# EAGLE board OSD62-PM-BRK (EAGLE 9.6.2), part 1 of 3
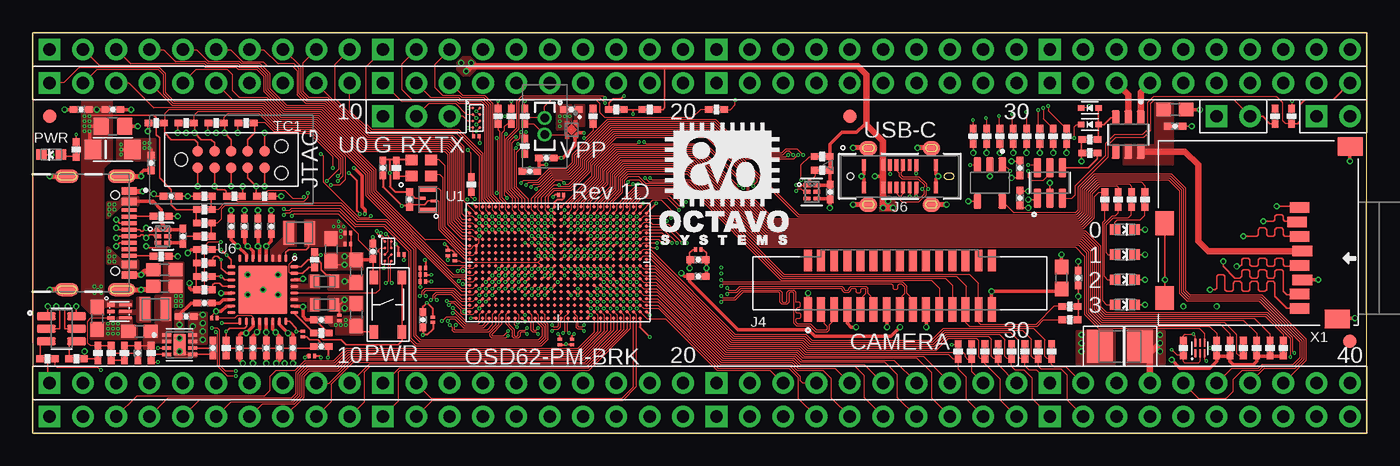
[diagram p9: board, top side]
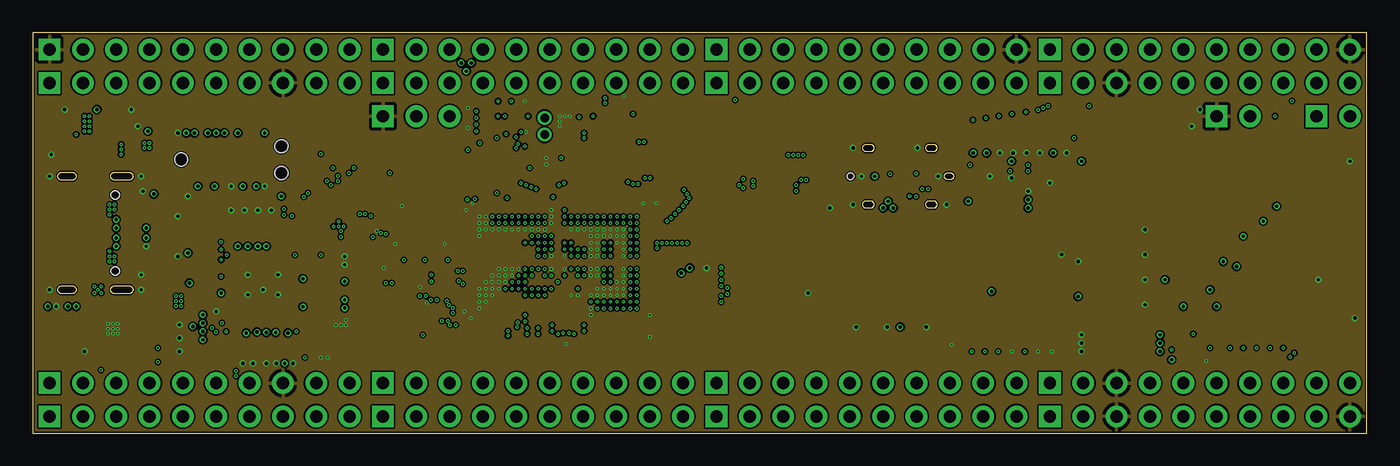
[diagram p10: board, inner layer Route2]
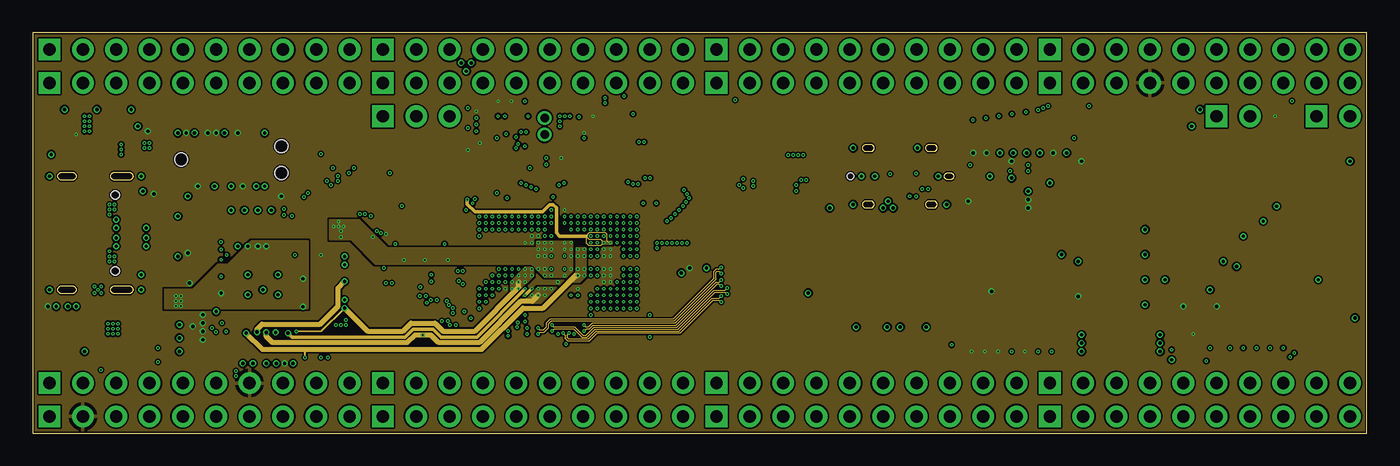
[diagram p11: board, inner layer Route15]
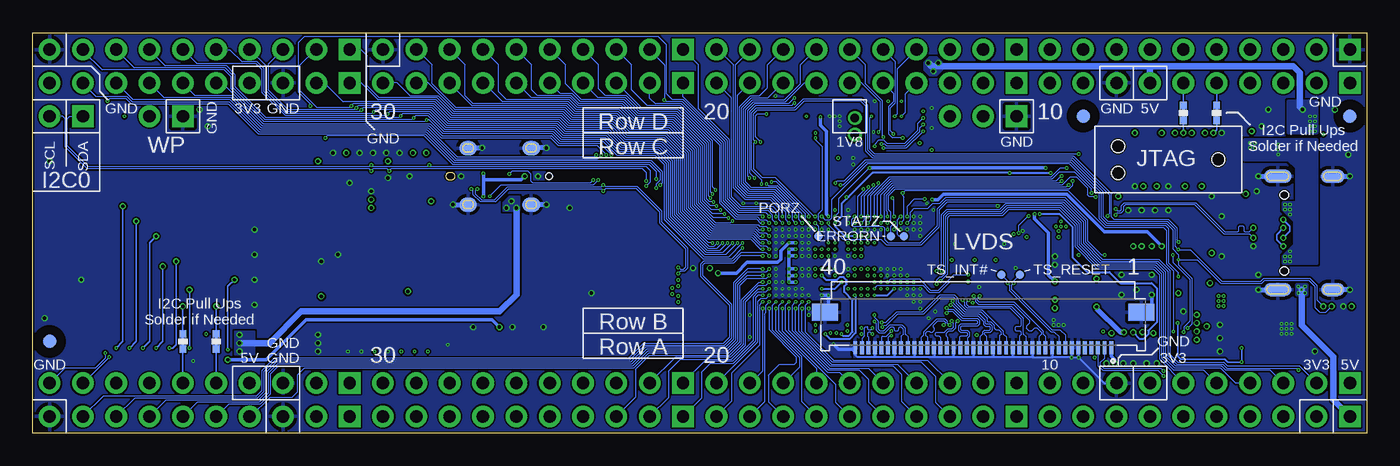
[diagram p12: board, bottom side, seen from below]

Size 101.6 x 30.48 mm. Coordinates in mm from the lower left corner, seen from the top.
Outline: 0,0 101.6,0 101.6,30.48 0,30.48 0,0
Copper layers (1+2*15+16): Top 0.035mm / dielectric 0.23mm / Route2 0.035mm / dielectric 0.93mm / Route15 0.035mm / dielectric 0.23mm / Bottom 0.035mm
Design rules "OSD32MP15x-BRK_Board_4lyr *": minimum track width 3mil, minimum drill 4mil, track to track 3mil, track to pad 3mil, pad to pad 3mil, via to via 3mil, smd to smd 3mil, copper to edge 5mil, drill to drill 4mil, minimum pad ring 3mil, minimum via ring 3mil, stop-mask expansion 3mil, vias tented up to drill 25mil, thermal gap 10mil

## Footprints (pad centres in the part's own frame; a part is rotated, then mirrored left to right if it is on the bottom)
C0201 = smd 0.23 x 0.34: 1 -0.205,0; 2 0.205,0
C0402 = smd 0.61 x 0.508: 1 -0.559,0; 2 0.559,0
B/3528-21R = smd 1.95 x 2.5: + 1.525,0; - -1.525,0
C0603 = smd 1.1 x 1: 1 -0.85,0; 2 0.85,0
C0805 = smd 1.143 x 1.27: 1 -0.889,0; 2 0.889,0
EIA-STD = smd 0.787 x 0.787: 1 -0.749,0; 2 0.749,0
RB520S30T1G = smd 0.48 x 0.4: ANODE 0.66,0; CATHODE -0.66,0
SOD-123FL = smd 1.25 x 1.5: A 1.5,0; C -1.5,0
FIDUCIAL_40MIL = smd 1.016 x 1.016: P$1 0,0
H1X2-1.27 = drill 0.65 pad 1.05: 1 -0.635,0; 2 0.635,0
H1X2-2.54 = drill 0.94 pad 1.651 square: 1 0,1.27 | drill 0.94 pad 1.651: 2 0,-1.27
TE_1-1734248-5 = smd 0.6 x 1.85: 1 -7,-2.025; 2 -6,-2.025; 3 -5,-2.025; 4 -4,-2.025; 5 -3,-2.025; 6 -2,-2.025; 7 -1,-2.025; 8 0,-2.025; 9 1,-2.025; 10 2,-2.025; 11 3,-2.025; 12 4,-2.025; 13 5,-2.025; 14 6,-2.025; 15 7,-2.025 | smd 0.6 x 1.65: 1_1 -7,1.725; 2_1 -6,1.725; 3_1 -5,1.725; 4_1 -4,1.725; 5_1 -3,1.725; 6_1 -2,1.725; 7_1 -1,1.725; 8_1 0,1.725; 9_1 1,1.725; 10_1 2,1.725; 11_1 3,1.725; 12_1 4,1.725; 13_1 5,1.725; 14_1 6,1.725; 15_1 7,1.725
GCT_USB4105-GF-A = smd 0.6 x 1.15: A1_B12 -3.2,4.755; A4_B9 -2.4,4.755; B1_A12 3.2,4.755; B4_A9 2.4,4.755 | smd 0.3 x 1.15: A5 -1.25,4.755; A6 -0.25,4.755; A7 0.25,4.755; A8 1.25,4.755; B5 1.75,4.755; B6 0.75,4.755; B7 -0.75,4.755; B8 -1.75,4.755 | smd 1 x 2.1 bottom: SH1_B -4.32,4.18; SH2_B 4.32,4.18 | smd 1 x 2.1: SH1_T -4.32,4.18; SH2_T 4.32,4.18 | smd 1 x 1.8 bottom: SH3_B 4.32,0; SH4_B -4.32,0 | smd 1 x 1.8: SH3_T 4.32,0; SH4_T -4.32,0 | hole 0.65: 2.89,3.68; -2.89,3.68
MOLEX_2171820001 = smd 0.3 x 0.87: A1 -2.75,0.865; A4 -1.25,0.865; A5 -0.75,0.865; A6 -0.25,0.865; A7 0.25,0.865; A8 0.75,0.865; A9 1.25,0.865; A12 2.75,0.865; B1 2.75,-0.865; B4 1.25,-0.865; B5 0.75,-0.865; B6 0.25,-0.865; B7 -0.25,-0.865; B8 -0.75,-0.865; B9 -1.25,-0.865; B12 -2.75,-0.865 | smd 1.35 x 1.1 bottom: SH_B_1 -2.4,2.15; SH_B_2 2.4,2.15; SH_B_3 2.4,-2.15; SH_B_4 -2.4,-2.15 | smd 1.35 x 1.1: SH_T_1 -2.4,2.15; SH_T_2 2.4,2.15; SH_T_3 2.4,-2.15; SH_T_4 -2.4,-2.15 | hole 0.52: -3.75,0
MOLEX_505110-4091 = smd 0.3 x 1: 1 -9.75,2.425; 2 -9.25,2.425; 3 -8.75,2.425; 4 -8.25,2.425; 5 -7.75,2.425; 6 -7.25,2.425; 7 -6.75,2.425; 8 -6.25,2.425; 9 -5.75,2.425; 10 -5.25,2.425; 11 -4.75,2.425; 12 -4.25,2.425; 13 -3.75,2.425; 14 -3.25,2.425; 15 -2.75,2.425; 16 -2.25,2.425; 17 -1.75,2.425; 18 -1.25,2.425; 19 -0.75,2.425; 20 -0.25,2.425; 21 0.25,2.425; 22 0.75,2.425; 23 1.25,2.425; 24 1.75,2.425; 25 2.25,2.425; 26 2.75,2.425; 27 3.25,2.425; 28 3.75,2.425; 29 4.25,2.425; 30 4.75,2.425; 31 5.25,2.425; 32 5.75,2.425; 33 6.25,2.425; 34 6.75,2.425; 35 7.25,2.425; 36 7.75,2.425; 37 8.25,2.425; 38 8.75,2.425; 39 9.25,2.425; 40 9.75,2.425 | smd 2 x 1.3: S1 -12.05,-0.275; S2 12.05,-0.275
H1X3-2.54 = drill 0.94 pad 1.651 square: 1 0,2.54 | drill 0.94 pad 1.651: 2 0,0; 3 0,-2.54
H1X40-2.54 = drill 0.94 pad 1.651 square: 1 0,49.53; 11 0,24.13; 21 0,-1.27; 31 0,-26.67 | drill 0.94 pad 1.651: 2 0,46.99; 3 0,44.45; 4 0,41.91; 5 0,39.37; 6 0,36.83; 7 0,34.29; 8 0,31.75; 9 0,29.21; 10 0,26.67; 12 0,21.59; 13 0,19.05; 14 0,16.51; 15 0,13.97; 16 0,11.43; 17 0,8.89; 18 0,6.35; 19 0,3.81; 20 0,1.27; 22 0,-3.81; 23 0,-6.35; 24 0,-8.89; 25 0,-11.43; 26 0,-13.97; 27 0,-16.51; 28 0,-19.05; 29 0,-21.59; 30 0,-24.13; 32 0,-29.21; 33 0,-31.75; 34 0,-34.29; 35 0,-36.83; 36 0,-39.37; 37 0,-41.91; 38 0,-44.45; 39 0,-46.99; 40 0,-49.53
L0806 = smd 0.8 x 1.8: 1 -0.8,0; 2 0.8,0
L0603 = smd 0.7 x 1: 1 -0.75,0; 2 0.75,0
R0402 = smd 0.61 x 0.508: 1 -0.559,0; 2 0.559,0
TACT4.2MM = smd 1.05 x 0.65: P$1 -2.075,1.075; P$2 2.075,1.075; P$3 -2.075,-1.075; P$4 2.075,-1.075
TC2050-IDC-NL = smd 0.787 x 0.787: 1 -2.54,-0.635; 2 -1.27,-0.635; 3 0,-0.635; 4 1.27,-0.635; 5 2.54,-0.635; 6 2.54,0.635; 7 1.27,0.635; 8 0,0.635; 9 -1.27,0.635; 10 -2.54,0.635 | hole 0.991: -3.81,0; 3.81,1.016; 3.81,-1.016
TP_B0,65 = smd 0.635 x 0.635: TP 0,0
BGA-500-9X14MM = smd 0.25 x 0.25: A2 -6.25,4.25; A3 -5.75,4.25; A4 -5.25,4.25; A5 -4.75,4.25; A6 -4.25,4.25; A7 -3.75,4.25; A8 -3.25,4.25; A9 -2.75,4.25; A10 -2.25,4.25; A11 -1.75,4.25; A12 -1.25,4.25; A13 -0.75,4.25; A14 -0.25,4.25; A15 0.25,4.25; A16 0.75,4.25; A17 1.25,4.25; A18 1.75,4.25; A19 2.25,4.25; A20 2.75,4.25; A21 3.25,4.25; A22 3.75,4.25; A23 4.25,4.25; A24 4.75,4.25; A25 5.25,4.25; A26 5.75,4.25; A27 6.25,4.25; B1 -6.75,3.75; B2 -6.25,3.75; B3 -5.75,3.75; B4 -5.25,3.75; B5 -4.75,3.75; B6 -4.25,3.75; B7 -3.75,3.75; B8 -3.25,3.75; B9 -2.75,3.75; B10 -2.25,3.75; B11 -1.75,3.75; B12 -1.25,3.75; B13 -0.75,3.75; B14 -0.25,3.75; B15 0.25,3.75; B16 0.75,3.75; B17 1.25,3.75; B18 1.75,3.75; B19 2.25,3.75; B20 2.75,3.75; B21 3.25,3.75; B22 3.75,3.75; B23 4.25,3.75; B24 4.75,3.75; B25 5.25,3.75; B26 5.75,3.75; B27 6.25,3.75; B28 6.75,3.75; C1 -6.75,3.25; C2 -6.25,3.25; C3 -5.75,3.25; C4 -5.25,3.25; C5 -4.75,3.25; C6 -4.25,3.25; C7 -3.75,3.25; C8 -3.25,3.25; C9 -2.75,3.25; C10 -2.25,3.25; C11 -1.75,3.25; C12 -1.25,3.25; C13 -0.75,3.25; C14 -0.25,3.25; C15 0.25,3.25; C16 0.75,3.25; C17 1.25,3.25; C18 1.75,3.25; C19 2.25,3.25; C20 2.75,3.25; C21 3.25,3.25; C22 3.75,3.25; C23 4.25,3.25; C24 4.75,3.25; C25 5.25,3.25; C26 5.75,3.25; C27 6.25,3.25; C28 6.75,3.25; D1 -6.75,2.75; D2 -6.25,2.75; D3 -5.75,2.75; D4 -5.25,2.75; D5 -4.75,2.75; D6 -4.25,2.75; D7 -3.75,2.75; D8 -3.25,2.75; D9 -2.75,2.75; D10 -2.25,2.75; D11 -1.75,2.75; D12 -1.25,2.75; D13 -0.75,2.75; D14 -0.25,2.75; D15 0.25,2.75; D16 0.75,2.75; D17 1.25,2.75; D18 1.75,2.75; D19 2.25,2.75; D20 2.75,2.75; D21 3.25,2.75; D22 3.75,2.75; D23 4.25,2.75; D24 4.75,2.75; D25 5.25,2.75; D26 5.75,2.75; D27 6.25,2.75; D28 6.75,2.75; E1 -6.75,2.25; E2 -6.25,2.25; E3 -5.75,2.25; E4 -5.25,2.25; E5 -4.75,2.25; E6 -4.25,2.25; E7 -3.75,2.25; E8 -3.25,2.25; E9 -2.75,2.25; E10 -2.25,2.25; E11 -1.75,2.25; E12 -1.25,2.25; E13 -0.75,2.25; E14 -0.25,2.25; E15 0.25,2.25; E16 0.75,2.25; E17 1.25,2.25; E18 1.75,2.25; E19 2.25,2.25; E20 2.75,2.25; E21 3.25,2.25; E22 3.75,2.25; E23 4.25,2.25; E24 4.75,2.25; E25 5.25,2.25; E26 5.75,2.25; E27 6.25,2.25; E28 6.75,2.25; F1 -6.75,1.75; F2 -6.25,1.75; F3 -5.75,1.75; F4 -5.25,1.75; F5 -4.75,1.75; F6 -4.25,1.75; F7 -3.75,1.75; F8 -3.25,1.75; F9 -2.75,1.75; F10 -2.25,1.75; F11 -1.75,1.75; F12 -1.25,1.75; F13 -0.75,1.75; F14 -0.25,1.75; F15 0.25,1.75; F16 0.75,1.75; F17 1.25,1.75; F18 1.75,1.75; F19 2.25,1.75; F20 2.75,1.75; F21 3.25,1.75; F22 3.75,1.75; F23 4.25,1.75; F24 4.75,1.75; F25 5.25,1.75; F26 5.75,1.75; F27 6.25,1.75; F28 6.75,1.75; G1 -6.75,1.25; G2 -6.25,1.25; G3 -5.75,1.25; G4 -5.25,1.25; G5 -4.75,1.25; G6 -4.25,1.25; G7 -3.75,1.25; G8 -3.25,1.25; G9 -2.75,1.25; G10 -2.25,1.25; G11 -1.75,1.25; G12 -1.25,1.25; G13 -0.75,1.25; G14 -0.25,1.25; G15 0.25,1.25; G16 0.75,1.25; G17 1.25,1.25; G18 1.75,1.25; G19 2.25,1.25; G20 2.75,1.25; G21 3.25,1.25; G22 3.75,1.25; G23 4.25,1.25; G24 4.75,1.25; G25 5.25,1.25; G26 5.75,1.25; G27 6.25,1.25; G28 6.75,1.25; H1 -6.75,0.75; H2 -6.25,0.75; H3 -5.75,0.75; H4 -5.25,0.75; H5 -4.75,0.75; H6 -4.25,0.75; H7 -3.75,0.75; H8 -3.25,0.75; H9 -2.75,0.75; H10 -2.25,0.75; H11 -1.75,0.75; H12 -1.25,0.75; H13 -0.75,0.75; H14 -0.25,0.75; H15 0.25,0.75; H16 0.75,0.75; H17 1.25,0.75; H18 1.75,0.75; H19 2.25,0.75; H20 2.75,0.75; H21 3.25,0.75; H22 3.75,0.75; H23 4.25,0.75; H24 4.75,0.75; H25 5.25,0.75; H26 5.75,0.75; H27 6.25,0.75; H28 6.75,0.75; J1 -6.75,0.25; J2 -6.25,0.25; J3 -5.75,0.25; J4 -5.25,0.25; J5 -4.75,0.25; J6 -4.25,0.25; J7 -3.75,0.25; J8 -3.25,0.25; J9 -2.75,0.25; J10 -2.25,0.25; J11 -1.75,0.25; J12 -1.25,0.25; J13 -0.75,0.25; J14 -0.25,0.25; J15 0.25,0.25; J16 0.75,0.25; J17 1.25,0.25; J18 1.75,0.25; J19 2.25,0.25; J20 2.75,0.25; J21 3.25,0.25; J22 3.75,0.25; J23 4.25,0.25; J24 4.75,0.25; J25 5.25,0.25; J26 5.75,0.25; J27 6.25,0.25; J28 6.75,0.25; K1 -6.75,-0.25; K2 -6.25,-0.25; K3 -5.75,-0.25; K4 -5.25,-0.25; K5 -4.75,-0.25; K6 -4.25,-0.25; K7 -3.75,-0.25; K8 -3.25,-0.25; K9 -2.75,-0.25; K10 -2.25,-0.25; K11 -1.75,-0.25; K12 -1.25,-0.25; K13 -0.75,-0.25; K14 -0.25,-0.25; K15 0.25,-0.25; K16 0.75,-0.25; K17 1.25,-0.25; K18 1.75,-0.25; K19 2.25,-0.25; K20 2.75,-0.25; K21 3.25,-0.25; K22 3.75,-0.25; K23 4.25,-0.25; K24 4.75,-0.25; K25 5.25,-0.25; K26 5.75,-0.25; K27 6.25,-0.25; K28 6.75,-0.25; L1 -6.75,-0.75; L2 -6.25,-0.75; L3 -5.75,-0.75; L4 -5.25,-0.75; L5 -4.75,-0.75; L6 -4.25,-0.75; L7 -3.75,-0.75; L8 -3.25,-0.75; L9 -2.75,-0.75; L10 -2.25,-0.75; L11 -1.75,-0.75; L12 -1.25,-0.75; L13 -0.75,-0.75; L14 -0.25,-0.75; L15 0.25,-0.75; L16 0.75,-0.75; L17 1.25,-0.75; L18 1.75,-0.75; L19 2.25,-0.75; L20 2.75,-0.75; L21 3.25,-0.75; L22 3.75,-0.75; L23 4.25,-0.75; L24 4.75,-0.75; L25 5.25,-0.75; L26 5.75,-0.75; L27 6.25,-0.75; L28 6.75,-0.75; M1 -6.75,-1.25; M2 -6.25,-1.25; M3 -5.75,-1.25; M4 -5.25,-1.25; M5 -4.75,-1.25; M6 -4.25,-1.25; M7 -3.75,-1.25; M8 -3.25,-1.25; M9 -2.75,-1.25; M10 -2.25,-1.25; M11 -1.75,-1.25; M12 -1.25,-1.25; M13 -0.75,-1.25; M14 -0.25,-1.25; M15 0.25,-1.25; M16 0.75,-1.25; M17 1.25,-1.25; M18 1.75,-1.25; M19 2.25,-1.25; M20 2.75,-1.25; M21 3.25,-1.25; M22 3.75,-1.25; M23 4.25,-1.25; M24 4.75,-1.25; M25 5.25,-1.25; M26 5.75,-1.25; M27 6.25,-1.25; M28 6.75,-1.25; N1 -6.75,-1.75; N2 -6.25,-1.75; N3 -5.75,-1.75; N4 -5.25,-1.75; N5 -4.75,-1.75; N6 -4.25,-1.75; N7 -3.75,-1.75; N8 -3.25,-1.75; N9 -2.75,-1.75; N10 -2.25,-1.75; N11 -1.75,-1.75; N12 -1.25,-1.75; N13 -0.75,-1.75; N14 -0.25,-1.75; N15 0.25,-1.75; N16 0.75,-1.75; N17 1.25,-1.75; N18 1.75,-1.75; N19 2.25,-1.75; N20 2.75,-1.75; N21 3.25,-1.75; N22 3.75,-1.75; N23 4.25,-1.75; N24 4.75,-1.75; N25 5.25,-1.75; N26 5.75,-1.75; N27 6.25,-1.75; N28 6.75,-1.75; P1 -6.75,-2.25; P2 -6.25,-2.25; P3 -5.75,-2.25; P4 -5.25,-2.25; P5 -4.75,-2.25; P6 -4.25,-2.25; P7 -3.75,-2.25; P8 -3.25,-2.25; P9 -2.75,-2.25; P10 -2.25,-2.25; P11 -1.75,-2.25; P12 -1.25,-2.25; P13 -0.75,-2.25; P14 -0.25,-2.25; P15 0.25,-2.25; P16 0.75,-2.25; P17 1.25,-2.25; P18 1.75,-2.25; P19 2.25,-2.25; P20 2.75,-2.25; P21 3.25,-2.25; P22 3.75,-2.25; P23 4.25,-2.25; P24 4.75,-2.25; P25 5.25,-2.25; P26 5.75,-2.25; P27 6.25,-2.25; P28 6.75,-2.25; R1 -6.75,-2.75; R2 -6.25,-2.75; R3 -5.75,-2.75; R4 -5.25,-2.75; R5 -4.75,-2.75; R6 -4.25,-2.75; R7 -3.75,-2.75; R8 -3.25,-2.75; R9 -2.75,-2.75; R10 -2.25,-2.75; R11 -1.75,-2.75; R12 -1.25,-2.75; R13 -0.75,-2.75; R14 -0.25,-2.75; R15 0.25,-2.75; R16 0.75,-2.75; R17 1.25,-2.75; R18 1.75,-2.75; R19 2.25,-2.75; R20 2.75,-2.75; R21 3.25,-2.75; R22 3.75,-2.75; R23 4.25,-2.75; R24 4.75,-2.75; R25 5.25,-2.75; R26 5.75,-2.75; R27 6.25,-2.75; R28 6.75,-2.75; T1 -6.75,-3.25; T2 -6.25,-3.25; T3 -5.75,-3.25; T4 -5.25,-3.25; T5 -4.75,-3.25; T6 -4.25,-3.25; T7 -3.75,-3.25; T8 -3.25,-3.25; T9 -2.75,-3.25; T10 -2.25,-3.25; T11 -1.75,-3.25; T12 -1.25,-3.25; T13 -0.75,-3.25; T14 -0.25,-3.25; T15 0.25,-3.25; T16 0.75,-3.25; T17 1.25,-3.25; T18 1.75,-3.25; T19 2.25,-3.25; T20 2.75,-3.25; T21 3.25,-3.25; T22 3.75,-3.25; T23 4.25,-3.25; T24 4.75,-3.25; T25 5.25,-3.25; T26 5.75,-3.25; T27 6.25,-3.25; T28 6.75,-3.25; U1 -6.75,-3.75; U2 -6.25,-3.75; U3 -5.75,-3.75; U4 -5.25,-3.75; U5 -4.75,-3.75; U6 -4.25,-3.75; U7 -3.75,-3.75; U8 -3.25,-3.75; U9 -2.75,-3.75; U10 -2.25,-3.75; U11 -1.75,-3.75; U12 -1.25,-3.75; U13 -0.75,-3.75; U14 -0.25,-3.75; U15 0.25,-3.75; U16 0.75,-3.75; U17 1.25,-3.75; U18 1.75,-3.75; U19 2.25,-3.75; U20 2.75,-3.75; U21 3.25,-3.75; U22 3.75,-3.75; U23 4.25,-3.75; U24 4.75,-3.75; U25 5.25,-3.75; U26 5.75,-3.75; U27 6.25,-3.75; U28 6.75,-3.75; V2 -6.25,-4.25; V3 -5.75,-4.25; V4 -5.25,-4.25; V5 -4.75,-4.25; V6 -4.25,-4.25; V7 -3.75,-4.25; V8 -3.25,-4.25; V9 -2.75,-4.25; V10 -2.25,-4.25; V11 -1.75,-4.25; V12 -1.25,-4.25; V13 -0.75,-4.25; V14 -0.25,-4.25; V15 0.25,-4.25; V16 0.75,-4.25; V17 1.25,-4.25; V18 1.75,-4.25; V19 2.25,-4.25; V20 2.75,-4.25; V21 3.25,-4.25; V22 3.75,-4.25; V23 4.25,-4.25; V24 4.75,-4.25; V25 5.25,-4.25; V26 5.75,-4.25; V27 6.25,-4.25
DRY6 = smd 0.55 x 0.3: 1 -0.355,0.5 | smd 0.52 x 0.3: 2 -0.37,0; 3 -0.37,-0.5; 4 0.37,-0.5; 5 0.37,0; 6 0.37,0.5
DMQ0006A = smd 0.6 x 0.25: 1 -0.65,0.5; 2 -0.65,0; 3 -0.65,-0.5 | smd 1 x 0.2: 4 0.45,-0.5; 5 0.45,0; 6 0.45,0.5
SOT95P280X145-5N = smd 1.1 x 0.6: 1 -1.4,0.95; 2 -1.4,0; 3 -1.4,-0.95; 4 1.4,-0.95; 5 1.4,0.95
SON50P200X200X80-9N = smd 0.76 x 0.28: 1 -0.985,0.75; 2 -0.985,0.25; 3 -0.985,-0.25; 4 -0.985,-0.75; 5 0.985,-0.75; 6 0.985,-0.25; 7 0.985,0.25; 8 0.985,0.75 | smd 0.9 x 1.6: 9 0,0
RHB0032W = smd 0.6 x 0.25: 1 -2.4,1.75; 2 -2.4,1.25; 3 -2.4,0.75; 4 -2.4,0.25; 5 -2.4,-0.25; 6 -2.4,-0.75; 7 -2.4,-1.25; 8 -2.4,-1.75; 17 2.4,-1.75; 18 2.4,-1.25; 19 2.4,-0.75; 20 2.4,-0.25; 21 2.4,0.25; 22 2.4,0.75; 23 2.4,1.25; 24 2.4,1.75 | smd 0.25 x 0.6: 9 -1.75,-2.4; 10 -1.25,-2.4; 11 -0.75,-2.4; 12 -0.25,-2.4; 13 0.25,-2.4; 14 0.75,-2.4; 15 1.25,-2.4; 16 1.75,-2.4; 25 1.75,2.4; 26 1.25,2.4; 27 0.75,2.4; 28 0.25,2.4; 29 -0.25,2.4; 30 -0.75,2.4; 31 -1.25,2.4; 32 -1.75,2.4 | smd 3.7 x 3.7: PAD 0,0
SOT95P280X110-6N = smd 1.45 x 0.59: 1 -1.155,0.95; 2 -1.155,0; 3 -1.155,-0.95; 4 1.155,-0.95; 5 1.155,0; 6 1.155,0.95
SOT95P280X145-6N = smd 1.1 x 0.6: 1 -1.3,0.95; 2 -1.3,0; 3 -1.3,-0.95; 4 1.3,-0.95; 5 1.3,0; 6 1.3,0.95
SON35P100X100X40-6N = smd 0.6 x 0.17: 1 -0.4,0.35; 2 -0.4,0; 3 -0.4,-0.35; 4 0.4,-0.35; 5 0.4,0; 6 0.4,0.35
YZP0008 = smd 0.23 x 0.23: A1 -0.25,0.75; A2 0.25,0.75; B1 -0.25,0.25; B2 0.25,0.25; C1 -0.25,-0.25; C2 0.25,-0.25; D1 -0.25,-0.75; D2 0.25,-0.75
DQN0004A = smd 0.05 x 0.05: 1 -0.43,0.325; 2 -0.43,-0.325; 3 0.43,-0.325; 4 0.43,0.325; 5 0,0
MF-MICROSD = smd 1.4 x 1.9: G0 -6.589,7.001; G1 6.561,6.001 | smd 0.8 x 1.5: PIN1 -1.939,3.151; PIN2 -0.839,2.951; PIN3 0.261,3.151; PIN4 1.361,3.351; PIN5 2.461,3.151; PIN6 3.561,3.351; PIN7 4.661,3.151; PIN8 5.761,3.151 | smd 1.8 x 1.4: PIN9 4.961,-7.149; PIN10 -0.739,-7.149
SIT1533AI_2X1.2MM = smd 0.4 x 1.4: 1 -0.8,0; 3 0.8,0 | smd 0.2 x 0.5: 2 -0.1,-0.45; 4 0.1,0.45
QFN-4-2X1.6MM = smd 0.9 x 0.8: 1 -0.75,-0.6; 2 0.75,-0.6; 3 0.75,0.6; 4 -0.75,0.6

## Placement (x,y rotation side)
C1  0.1uF  [C0201]  30.48,8.64 90 top
C2  0.1uF  [C0201]  41.07,6.93 270 top
C3  0.1uF  [C0201]  40.23,18.14 0 top
C4  1uF  [C0402]  29.72,8.64 90 top
C5  4.7uF  [C0402]  21.97,6.6 0 top
C6  0.1uF  [C0201]  50.67,13.97 0 top
C7  0.1uF  [C0201]  23.37,8.76 270 top
C8  0.1uF  [C0201]  29.72,12.06 180 top
C9  0.1uF  [C0201]  20.57,7.54 270 top
C10  0.1uF  [C0201]  31.62,13.72 90 top
C11  0.1uF  [C0201]  24,15.24 0 top
C12  0.1uF  [C0201]  28.07,13.59 180 top
C13  0.1uF  [C0201]  32.13,13.34 90 top
C14  0.1uF  [C0201]  24,14.4 0 top
C15  0.1uF  [C0201]  29.72,12.57 180 top
C16  10uF  [C0402]  25.91,13.84 270 top
C17  0.1uF  [C0201]  21.26,5.87 0 top
C18  0.1uF  [C0201]  13.84,8.76 180 top
C19  0.1uF  [C0201]  40.16,6.93 270 top
C20  0.1uF  [C0201]  29.72,11.56 180 top
C21  2.2uF  [C0402]  37.85,19.94 0 top
C22  2.2uF  [C0402]  50.67,13.21 0 top
C23  2.2uF  [C0402]  50.67,11.94 0 top
C24  0.1uF  [C0402]  60.73,18.36 270 top
C25  220uF  [B/3528-21R]  82.8,6.6 0 top
C26  0.1uF  [C0402]  75.18,17.91 90 top
C27  10uF  [C0603]  4.9,8.74 270 top
C28  DNP  [C0402]  13.72,6.48 270 top
C29  0.1uF  [C0402]  11.68,8.89 180 top
C30  120pF  [C0402]  8,6.1 90 top
C31  10uF  [C0603]  10.03,11.18 180 top
C32  10uF  [C0603]  10.03,12.45 180 top
C33  10uF  [C0603]  8.13,7.75 180 top
C34  0.1uF  [C0402]  10.54,18.03 0 top
C35  0.1uF  [C0402]  75.18,20.19 270 top
C36  0.1uF  [C0402]  79.63,11.81 90 top
C37  10uF  [C0603]  78.36,11.81 90 top
C38  10uF  [C0402]  16.76,6.48 270 top
C39  10uF  [C0402]  18.8,6.48 270 top
C40  10uF  [C0402]  16.13,15.75 90 top
C41  2.2uF  [C0402]  13.08,9.91 180 top
C42  10uF  [C0402]  15.11,15.75 90 top
C43  10uF  [C0402]  15.75,6.48 270 top
C44  10uF  [C0402]  17.78,6.48 270 top
C45  10uF  [C0402]  19.81,6.48 270 top
C46  0.1uF  [C0402]  28.7,17.78 270 top
C47  47uF  [C0603]  24.64,9.02 270 top
C48  22uF  [C0402]  21.97,8.64 0 top
C49  47uF  [C0603]  24.64,12.32 90 top
C50  0.1uF  [C0402]  11.43,14.99 270 top
C51  10uF  [C0402]  17.14,15.75 90 top
C52  22uF  [C0402]  18.16,15.75 90 top
C53  47uF  [C0603]  22.73,13.97 270 top
C54  0.1uF  [C0402]  26.67,20.19 270 top
C55  0.1uF  [C0402]  6.1,24.64 0 top
C56  47uF  [C0805]  6.1,23.37 0 top
C57  10uF  [C0603]  87,24.64 0 top
C58  0.1uF  [C0402]  87,23.37 0 top
C59  1nF  [C0402]  3.68,24.64 180 top
C60  4.7uF  [C0402]  9.02,20.57 270 top
C61  0.1uF  [C0201]  33.78,22.61 180 top
C62  1uF  [C0402]  41.02,24.64 180 top
C63  1uF  [C0402]  39.12,20.95 180 top
D1  RED  [EIA-STD]  1.4,21.21 180 top
D2  GREEN  [EIA-STD]  83.19,11.68 0 top
D3  GREEN  [EIA-STD]  83.19,9.78 0 top
D4  GREEN  [EIA-STD]  83.19,13.59 0 top
D5  GREEN  [EIA-STD]  83.19,15.49 0 top
D6  RB520S30T1G  [RB520S30T1G]  80.52,23.5 0 top
D7  RB520S30T1G  [RB520S30T1G]  80.52,24.77 0 top
D8  RBS2MM40C  [SOD-123FL]  6.1,21.59 0 top
FUD1  FIDUCIAL  [FIDUCIAL_40MIL]  100.33,6.99 0 top
FUD2  FIDUCIAL  [FIDUCIAL_40MIL]  1.27,24.13 90 top
FUD3  FIDUCIAL  [FIDUCIAL_40MIL]  1.27,24.13 90 bottom
FUD4  FIDUCIAL  [FIDUCIAL_40MIL]  100.33,6.99 0 bottom
FUD5  FIDUCIAL  [FIDUCIAL_40MIL]  21.59,24.13 90 bottom
FUD6  FIDUCIAL  [FIDUCIAL_40MIL]  62.23,24.13 90 top
J1  [H1X2-1.27]  38.99,23.37 270 top
J2  [H1X2-2.54]  91.44,24.13 90 top
J4  1-1734248-5  [TE_1-1734248-5]  66.04,11.43 0 top
J5  USB4105-GF-A  [GCT_USB4105-GF-A]  2.6,15.24 270 top
J6  2171820001  [MOLEX_2171820001]  66.04,19.56 0 top
J7  [H1X2-2.54]  99.06,24.13 90 top
J8  505110-4091  [MOLEX_505110-4091]  29.21,8.92 180 bottom
JP1  [H1X3-2.54]  29.21,24.13 90 top
JP2  [H1X40-2.54]  50.8,1.27 90 top
JP3  [H1X40-2.54]  50.8,3.81 90 top
JP4  [H1X40-2.54]  50.8,26.67 90 top
JP5  [H1X40-2.54]  50.8,29.21 90 top
L1  0.47uH  [L0806]  9.35,9.45 0 top
L2  0.47uH  [L0603]  22.23,9.78 0 top
L3  0.47uH  [L0603]  22.23,11.56 0 top
L4  0.47uH  [L0806]  20.32,15.24 0 top
R1  10k  [R0402]  44.45,24.64 0 top
R2  100k  [R0402]  46.99,24.64 0 top
R3  10k  [R0402]  37.47,24.13 270 top
R4  10k  [R0402]  13.08,14.99 180 top
R5  20k  [R0402]  13.08,16 180 top
R6  100k  [R0402]  4.95,6.1 90 top
R7  10k  [R0402]  94.61,24.13 90 top
R8  270k  [R0402]  5.97,6.1 90 top
R9  180k  [R0402]  6.99,6.1 270 top
R10  10k  [R0402]  33.4,18.92 90 top
R11  10k  [R0402]  42.67,24.13 90 top
R12  2k  [R0402]  78.99,9.65 0 top
R13  10k  [R0402]  13.08,10.92 180 top
R14  10k  [R0402]  11.68,23.62 0 top
R15  10k  [R0402]  3.33,5.66 180 top
R16  10k  [R0402]  80.52,21.34 180 top
R17  10k  [R0402]  13.97,23.62 180 top
R18  10k  [R0402]  15.37,18.03 0 top
R19  10k  [R0402]  17.65,18.03 0 top
R20  10k  [R0402]  16.26,23.62 180 top
R21  10k  [R0402]  9.4,23.62 180 top
R22  10k  [R0402]  21.97,7.62 0 top
R23  10k  [R0402]  21.46,13.21 90 top
R24  10k  [R0402]  14.73,6.48 270 top
R25  10k  [R0402]  13.08,11.94 180 top
R26  10k  [R0402]  77.6,6.22 90 top
R27  10k  [R0402]  76.58,6.22 90 top
R28  10k  [R0402]  75.56,6.22 90 top
R29  10k  [R0402]  74.55,6.22 90 top
R30  10k  [R0402]  73.53,6.22 90 top
R31  10k  [R0402]  72.52,6.22 90 top
R32  10k  [R0402]  71.5,6.22 90 top
R33  22  [R0402]  92.2,6.48 270 top
R34  10k  [R0402]  70.48,6.22 90 top
R35  5.1K  [R0402]  9.78,16.51 180 top
R36  5.1K  [R0402]  9.78,13.46 180 top
R37  10k  [R0402]  78.74,22.61 270 top
R38  10k  [R0402]  77.72,22.61 270 top
R39  10k  [R0402]  76.71,22.61 270 top
R40  10k  [R0402]  75.69,22.61 270 top
R41  10k  [R0402]  74.68,22.61 270 top
R42  10k  [R0402]  73.66,22.61 270 top
R43  10k  [R0402]  95.25,6.48 270 top
R44  10k  [R0402]  94.23,6.48 270 top
R45  10k  [R0402]  93.22,6.48 270 top
R46  10k  [R0402]  91.19,6.48 270 top
R47  10k  [R0402]  90.17,6.48 270 top
R48  10k  [R0402]  87.63,6.48 90 top
R49  10k  [R0402]  72.64,22.61 270 top
R50  10k  [R0402]  27.69,20.19 270 top
R51  10k  [R0402]  71.63,22.61 270 top
R52  4.7k  [R0402]  13.08,12.95 180 top
R53  4.7k  [R0402]  13.08,13.97 180 top
R54  10k  [R0402]  80.52,22.35 0 top
R55  0  [R0402]  95.89,24.13 270 top
R56  0  [R0402]  1.12,5.66 180 top
R57  1k  [R0402]  3.3,21.59 90 top
R58  1k  [R0402]  82.68,17.78 90 top
R59  1k  [R0402]  81.66,17.78 90 top
R60  1k  [R0402]  83.69,17.78 90 top
R61  1k  [R0402]  84.71,17.78 90 top
R62  20k  [R0402]  13.08,17.02 180 top
R63  10k  [R0402]  13.08,18.03 180 top
R64  2k  [R0402]  78.99,8.64 0 top
R65  2k  [R0402]  36.45,24.13 90 top
R66  2k  [R0402]  35.43,24.13 90 top
R67  DNP  [R0402]  11.43,24.38 270 bottom
R68  DNP  [R0402]  13.97,24.38 270 bottom
R69  DNP  [R0402]  90.17,6.99 90 bottom
R70  DNP  [R0402]  87.63,6.99 90 bottom
R71  56K  [R0402]  60.12,21.06 0 top
R72  56K  [R0402]  60.12,20.02 0 top
R73  10k  [R0402]  9.02,6.1 90 top
R74  0  [R0402]  52.07,24.64 0 top
R76  10k  [R0402]  37.47,21.84 270 top
S1  MF-SW-TACT-4.2MM  [TACT4.2MM]  27.05,9.78 270 top
TC1  TC2050-IDC-NL  [TC2050-IDC-NL]  15.11,20.83 0 top
TP1  TPB0,65  [TP_B0,65]  41.75,15 90 bottom
TP2  TPB0,65  [TP_B0,65]  36.25,15 90 bottom
TP3  TPB0,65  [TP_B0,65]  35.25,15 90 bottom
TP6  TPB0,65  [TP_B0,65]  26.42,12.06 0 bottom
TP7  TPB0,65  [TP_B0,65]  27.81,12.06 0 bottom
U1  OSD6254-1G-BPM-ES  [BGA-500-9X14MM]  40,13 0 top
U2  TPD4S012_DRY_6_P1_P  [DRY6]  59.33,18.36 0 top
U3  TLV62595DMQR  [DMQ0006A]  6.6,9.27 0 top
U4  24AA32AT-I/OT  [SOT95P280X145-5N]  72.9,19.05 270 top
U5  TPS22965DSGT  [SON50P200X200X80-9N]  11.18,6.73 0 top
U6  TPS6521903RHB  [RHB0032W]  17.53,10.92 270 top
U7  ADC121C027CIMK  [SOT95P280X110-6N]  2.18,7.95 0 top
U8  ADC121C027CIMK  [SOT95P280X110-6N]  77.47,19.05 90 top
U9  TPD4S012_DRY_6_P1_P  [DRY6]  9.91,14.99 0 top
U10  TPS22918DBVR  [SOT95P280X145-6N]  83.44,22.73 270 top
U11  SN74LVC1G04DSFR  [SON35P100X100X40-6N]  88.9,6.48 90 top
U12  SN74LVC2G241YZPR  [YZP0008]  33.78,24 0 top
U13  SN74LVC2G241YZPR  [YZP0008]  27.05,13.84 0 top
U14  TLV75518PDQNR  [DQN0004A]  41.02,23.11 270 top
U$1  [OCTAVO-LOGO-8VO]  48.13,17.27 0 top
U$2  [OCTAVO-LOGO-WORDS-SMALL]  47.62,14.22 0 top
X1  MF-MICROSD  [MF-MICROSD]  93.34,15.24 270 top
Y1  SIT1533AI-H4-D14-32.768  [SIT1533AI_2X1.2MM]  30.1,17.78 90 top
Y2  SIT8008BI-73-YYS-25.000000  [QFN-4-2X1.6MM]  29.59,20.19 0 top

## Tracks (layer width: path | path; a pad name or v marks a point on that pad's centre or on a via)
3V3_FB
  Top 0.076: R6.2 4.39,6.66 4.19,6.86 4.19,8.53 4.43,8.77 U3.3
  Top 0.127: R6.2 R8.2 5.97,6.22 6.1,6.1 7.87,6.1 8,5.97 C30.1
3V3_FB_0
  Top 0.127: R8.1 R9.2
3V3_SW
  pour Top (no thermals): 6.6,9.27 8,9.27 8,10.29 8.89,10.29 8.89,8.51 8,8.51 8,9.14 6.6,9.14
ADC0_ADDR
  Top 0.127: R15.2 2.77,6.83 2.94,7 U7.4
ADC1_ADDR
  Top 0.127: U8.4 80.4,20.2 81.08,20.88 R16.1
BUCK1-0P75  (via drill 0.1 pad 0.25)
  Top 0.076: C13.1 32.51,13.13 32.64,13 38.5,13 | 38.5,13 U1.K12 | U1.J12 38.5,13
  Top 0.127: U6.1 19.28,13.78 19.47,13.97 20.83,13.97 20.99,14.13 20.99,15.11 L4.2 | C10.1 v31.62,13.18
  Top 0.152: U1.K12 v38.5,12.5 | U1.K13 v39,12.5 | U1.L13 v39,12 U1.M12 | U1.L14 v39.5,12 U1.M13 | U1.L15 v40.5,12 | U1.K16 v41,12.5 | U1.G12 v38.5,14.5 | U1.H12 v38.5,14 | U1.J12 v38.5,13.5 | U1.J13 v39,13.5 | U1.H13 v39,14 | U1.G14 v39.5,14.5 | U1.H14 v39.5,14 | U1.H15 v40.5,14 | U1.G15 v40.5,14.5 | U1.H16 v41,14 | U1.J16 v41,13.5 | U1.G16 v41,14.5 | U1.G13 v39,14.5 | C15.1 29.92,13.13 v29.87,13.18 | C12.1 v28.27,13.18
  Top 0.254: C16.1 v25.91,14.94
  other vias: 23.67,15.72 23.47,15.39 22.91,15.72 23.29,15.72 23.47,14.94 23.29,16.1
  pour Top (no thermals): 20.7,14.22 20.7,16.26 23.24,16.26 23.88,15.62 23.88,14.22
  pour Route15: 41.12,14.62 41.12,12.38 40.62,11.88 39,11.88 38,12.88 26.12,12.88 24.27,14.73 22.61,14.73 22.61,16.26 24.87,16.26 27,14.12 38.38,14.12 38.38,14.62
BUCK2-1P8  (via drill 0.1 pad 0.25, 0.25 pad 0.46)
  Top 0.076: U1.C15 v40.5,16.5
  Top 0.127: L3.2 22.98,11.7 22.61,12.06 22.35,12.06 21.97,12.45 21.97,12.95 21.72,13.21 20.95,13.21 20.42,12.67 U6.32
  Top 0.254: C38.1 16.76,7.37 17.07,7.67 v17.07,7.7 17.28,7.9 U6.20 | v24.46,20.19 25.07,19.58 25.07,17.22 25.3,16.99 v25.3,16.69 | C49.1 24.55,11.56 v23.75,11.56 | C21.1 37.72,19.94 37.85,20.07 v37.85,20.19
  Route15 0.381: v17.07,7.7 17.07,7.93 17.45,8.31 21.89,8.31 23.24,9.65 23.24,11.05 v23.75,11.56
  Bottom 0.076: v37.85,20.19 37.87,20.19 40.23,17.83 40.23,16.77 v40.5,16.5
  Bottom 0.254: v37.85,20.19 v24.46,20.19 | v23.75,11.56 24.23,12.04 24.23,15.24 25.3,16.31 v25.3,16.69
  pour Top (no thermals): 22.48,10.92 25.15,10.92 25.15,12.06 22.48,12.06
BUCK3-1P2  (via drill 0.1 pad 0.25, 0.25 pad 0.46)
  Top 0.127: U6.24 19.55,8.52 20.07,8 v20.07,7.75 C9.1
  Top 0.152: U1.M8 v36.5,11.5 | U1.N8 v36.5,11 | U1.N9 v37,11 | U1.M10 v37.5,11.5 | U1.M9 v37,11.5 | U1.L10 v37.5,12 | U1.L11 v38,12 | U1.K11 v38,12.5 | U1.L9 v37,12 | U1.K10 v37.5,12.5 | C7.1 23.37,9.78 v23.75,10.16 | C8.1 v30.35,12.06
  Route15 0.127: v20.07,7.75 21.97,7.75 v23.75,9.53
  Route15 0.381: v23.75,9.53 25.5,7.77 28.19,7.77 28.8,8.38 30.63,8.38 31.24,7.77 33.68,7.77 37,11.09 v37,11.5
  Bottom 0.076: v36.5,11.5 36.25,11.75 34.08,11.75 33.22,10.9 32.61,10.9 31.45,12.06 v30.35,12.06
  pour Top (no thermals): 22.48,10.41 25.15,10.41 25.15,9.27 22.48,9.27
  pour Route15 (rank 2): 36.38,11.5 37.5,12.62 38.12,12.62 38.12,12 37,10.88 36.38,10.88
CH1_LVDS_A0N  (via drill 0.1 pad 0.25)
  Top 0.076: U1.P2 33.5,10.5 32.63,10.5 32.08,11.05 29.87,11.05 29.64,10.82 29.64,10.59 v29.49,10.44
  Bottom 0.076: v29.49,10.44 29.64,10.29 29.64,10.13 29.49,9.98 26.82,9.98 24.61,7.77 24.61,7.54 24.46,7.39 J8.11
CH1_LVDS_A0P  (via drill 0.1 pad 0.25)
  Top 0.076: U1.R1 32.65,10.25 32,10.9 29.95,10.9 29.79,10.74 29.79,10.59 v29.95,10.44
  Bottom 0.076: v29.95,10.44 29.79,10.29 29.79,10.06 29.57,9.83 26.9,9.83 25.68,8.61 25.68,8.38 25.91,8.15 25.91,8 25.68,7.77 25.53,7.77 25.3,8 25.07,8 24.77,7.7 24.77,7.54 24.96,7.35 J8.12
CH1_LVDS_A1N  (via drill 0.1 pad 0.25)
  Top 0.076: U1.R2 33.5,10 32.67,10 31.93,10.74 30.71,10.74 30.48,10.52 30.48,10.29 v30.33,10.13
  Bottom 0.076: v30.33,10.13 30.48,9.98 30.48,9.83 30.33,9.68 27.05,9.68 26.14,8.76 26.14,7.54 25.96,7.37 J8.14
CH1_LVDS_A1P  (via drill 0.1 pad 0.25)
  Top 0.076: U1.T1 32.69,9.75 31.85,10.59 30.79,10.59 30.63,10.44 30.63,10.29 v30.79,10.13
  Bottom 0.076: v30.79,10.13 30.63,9.98 30.63,9.75 30.4,9.53 27.13,9.53 26.29,8.69 26.29,8.23 26.36,8.15 26.67,8.15 26.75,8.08 26.75,7.85 26.67,7.77 26.36,7.77 26.29,7.7 26.29,7.54 26.46,7.37 J8.15
CH1_LVDS_A2N  (via drill 0.1 pad 0.25)
  Top 0.076: U1.T2 33.5,9.5 32.72,9.5 32.16,10.06 v31.55,10.06
  Bottom 0.076: v31.55,10.06 31.55,9.98 30.63,9.07 29.49,9.07 29.03,8.61 29.03,8.38 28.96,8.31 28.65,8.31 28.5,8.15 28.5,7.85 28.65,7.7 29.03,7.7 29.11,7.62 29.11,7.54 28.96,7.39 J8.20
CH1_LVDS_A2P  (via drill 0.1 pad 0.25)
  Top 0.076: U1.U2 33.5,9 32.76,9 32.61,9.14 32.61,9.37 32.08,9.91 31.85,9.91 v31.7,9.75
  Bottom 0.076: v31.7,9.75 31.55,9.75 30.71,8.91 29.57,8.91 29.18,8.53 29.18,8.31 29.03,8.15 28.73,8.15 28.65,8.08 28.65,7.92 28.73,7.85 29.11,7.85 29.26,7.7 29.26,7.54 29.46,7.34 J8.21
CH1_LVDS_A3N  (via drill 0.1 pad 0.25)
  Top 0.076: U1.U3 34,9 34,8.62 33.83,8.46 33.07,8.46 v32,9.53
  Bottom 0.076: v32,9.53 31.93,9.45 31.47,9.45 30.79,8.76 29.64,8.76 29.49,8.61 29.49,8.31 29.64,8.15 30.86,8.15 30.94,8.08 30.94,7.92 30.86,7.85 30.4,7.85 30.25,7.7 30.25,7.39 30.4,7.24 30.4,6.55 J8.23
CH1_LVDS_A3P  (via drill 0.1 pad 0.25)
  Top 0.076: U1.V3 34.25,8.65 33.91,8.31 32.99,8.31 32.16,9.14 v32,9.14
  Bottom 0.076: v32,9.14 31.85,9.3 31.55,9.3 30.86,8.61 29.72,8.61 29.64,8.53 29.64,8.38 29.72,8.31 30.94,8.31 31.09,8.15 31.09,7.85 30.94,7.7 30.48,7.7 30.4,7.62 30.4,7.47 30.48,7.39 30.94,7.39 31.01,7.32 31.01,6.54 J8.24
CH1_LVDS_CLKN  (via drill 0.1 pad 0.25)
  Top 0.076: v36.94,8.43 36.94,8.61 37,8.66 37,9 U1.U8
  Bottom 0.076: v36.94,8.43 36.6,8.43 35.81,9.22 33.83,9.22 32.54,10.52 31.37,10.52 31.09,10.23 31.09,9.98 30.48,9.37 29.26,9.37 27.66,7.77 27.66,7.54 27.46,7.34 J8.17
CH1_LVDS_CLKP  (via drill 0.1 pad 0.25)
  Top 0.076: U1.V8 36.75,8.58 36.65,8.48 36.65,8.31 v36.88,8.08
  Bottom 0.076: v36.88,8.08 36.73,8.23 36.58,8.23 35.74,9.07 33.76,9.07 32.46,10.36 31.43,10.36 31.24,10.17 31.24,9.91 30.56,9.22 29.34,9.22 28.88,8.76 28.88,8.53 28.8,8.46 28.57,8.46 28.35,8.23 28.35,8 28.19,7.85 27.96,7.85 27.81,7.7 27.81,7.54 27.96,7.4 J8.18
CH2_LVDS_A0N  (via drill 0.1 pad 0.25)
  Top 0.076: U1.U4 34.5,9 34.5,8.44 34.21,8.15 32.92,8.15 32.23,8.84 31.47,8.84 v31.17,8.53
  Bottom 0.076: v31.17,8.53 31.32,8.38 31.32,8 31.55,7.77 31.85,7.77 32,7.62 32,7.39 31.88,7.27 31.88,6.57 J8.26
CH2_LVDS_A0P  (via drill 0.1 pad 0.25)
  Top 0.076: U1.V4 34.75,8.46 34.29,8 32.84,8 32.16,8.69 31.77,8.69 v31.62,8.53
  Bottom 0.076: v31.62,8.53 31.47,8.38 31.47,8.08 31.62,7.92 31.93,7.92 32.16,7.7 32.77,7.7 32.84,7.62 32.84,7.47 32.77,7.39 32.53,7.39 32.46,7.32 J8.27
CH2_LVDS_A1N  (via drill 0.1 pad 0.25)
  Top 0.076: U1.U5 35,9 35,8.25 34.6,7.85 32.16,7.85 32.08,7.92 32.08,8.08 v32.23,8.23
  Bottom 0.076: v32.23,8.23 32.08,8.38 32.08,8.46 32.16,8.53 32.69,8.53 32.99,8.23 32.99,8.08 32.92,8 32.92,7.85 33.07,7.7 33.22,7.7 33.3,7.77 33.45,7.77 33.6,7.62 33.6,7.47 33.46,7.32 J8.29
CH2_LVDS_A1P  (via drill 0.1 pad 0.25)
  Top 0.076: U1.V5 35.25,8.25 34.7,7.7 32.08,7.7 31.93,7.85 31.93,8.08 v31.77,8.23
  Bottom 0.076: v31.77,8.23 31.93,8.38 31.93,8.53 32.08,8.69 32.77,8.69 33.76,7.7 33.76,7.47 33.96,7.26 J8.30
CH2_LVDS_A2N  (via drill 0.1 pad 0.25)
  Top 0.076: U1.U6 35.5,9 35.5,8.28 34.82,7.61 34.82,7.39 34.98,7.24 36.02,7.24 v36.2,7.42
  Bottom 0.076: v36.2,7.42 36.32,7.42 36.46,7.28 J8.35
CH2_LVDS_A2P  (via drill 0.1 pad 0.25)
  Top 0.076: v36.2,7.77 35.81,7.39 35.05,7.39 34.98,7.47 34.98,7.54 35.75,8.32 U1.V6
  Bottom 0.076: v36.2,7.77 36.58,7.39 36.88,7.39 36.96,7.31 J8.36
CH2_LVDS_A3N  (via drill 0.1 pad 0.25)
  Top 0.076: U1.U7 36,9 36,8.35 36.5,7.85 36.5,7.39 36.65,7.24 36.96,7.24 37.11,7.39 37.11,7.62 37.19,7.7 37.49,7.7 v37.64,7.54
  Bottom 0.076: v37.64,7.54 37.8,7.7 37.95,7.7 38.02,7.62 38.02,7.39 37.96,7.33 J8.38
CH2_LVDS_A3P  (via drill 0.1 pad 0.25)
  Top 0.076: U1.V7 36.25,8.33 36.65,7.92 36.65,7.47 36.73,7.39 36.88,7.39 36.96,7.47 36.96,7.7 37.11,7.85 37.49,7.85 v37.64,8
  Bottom 0.076: v37.64,8 37.8,7.85 37.9,7.85 37.97,7.92 37.97,8.05 38.04,8.12 38.16,8.12 38.24,8.04 38.24,7.4 38.46,7.18 J8.39
CH2_LVDS_CLKN  (via drill 0.1 pad 0.25)
  Top 0.076: U1.U9 v37.5,9
  Bottom 0.076: v37.5,9 37.5,8.84 37.19,8.53 37.19,7.92 37.03,7.77 36.8,7.77 36.35,8.23 35.37,8.23 35.13,7.99 35.13,7.54 34.96,7.38 J8.32
CH2_LVDS_CLKP  (via drill 0.1 pad 0.25)
  Top 0.076: U1.V9 v37.5,8.5
  Bottom 0.076: v37.5,8.5 37.34,8.34 37.34,7.85 37.11,7.62 36.73,7.62 36.27,8.08 36.04,8.08 35.97,8 35.97,7.86 35.88,7.77 35.75,7.77 35.66,7.86 35.66,8 35.59,8.08 35.43,8.08 35.28,7.92 35.28,7.54 35.46,7.36 J8.33
CLICK0_AN
  Top 0.127: JP3.1 1.14,3.94 1.14,5.38 0.86,5.66 R56.2 0.56,6.81 0.51,6.86 0.65,7 U7.3
CLICK1_AN
  Top 0.076: U8.3 79.16,17.89 79.4,18.14 79.4,18.82 81.69,21.11 81.69,22.02 82.37,22.71 84.51,22.71 84.89,23.09 84.89,25.15 85.34,25.6 94.77,25.6 95.22,25.15 95.22,23.77 95.43,23.57 R55.2
  Top 0.127: R55.2 96.34,23.57 96.52,23.75 96.52,25.02 96.9,25.4 99.06,25.4 JP4.40
CSI0_RXCLKN  (via drill 0.1 pad 0.25)
  Top 0.076: J4.8 66.22,9.58 66.22,10.44 66.45,10.67 66.45,11.12 66.22,11.35 65.99,11.35 65.91,11.28 65.91,11.05 65.84,10.97 65.61,10.97 65.53,11.05 65.53,11.28 65.46,11.35 52.58,11.35 v52.43,11.2 | v41.99,7.77 41.83,7.92 41.53,7.92 41.38,8.08 41.38,8.46 41.25,8.59 U1.V17
  Route15 0.076: v52.43,11.2 52.27,11.35 52.12,11.35 49,8.23 42.67,8.23 42.37,7.92 42.14,7.92 v41.99,7.77
CSI0_RXCLKP  (via drill 0.1 pad 0.25)
  Top 0.076: J4.9 66.83,9.62 66.83,10.44 66.6,10.67 66.6,11.2 66.29,11.51 52.58,11.51 v52.43,11.66 | v41.99,8.23 41.83,8.08 41.6,8.08 41.53,8.15 41.53,8.53 41.5,8.56 41.5,8.85 41.25,9.1 U1.U17
  Route15 0.076: v52.43,11.66 52.27,11.51 52.05,11.51 48.92,8.38 42.6,8.38 42.29,8.08 42.14,8.08 v41.99,8.23
CSI0_RXN0  (via drill 0.1 pad 0.25)
  Top 0.076: J4.2 60.27,9.17 60.27,8.38 60.5,8.15 60.5,7.92 60.43,7.85 59.74,7.85 59.28,8.31 58.29,8.31 58.14,8.46 58.14,8.69 58.22,8.76 58.45,8.76 58.52,8.84 58.52,9.07 58.45,9.14 58.22,9.14 58.14,9.22 58.14,9.45 58.27,9.58 58.41,9.58 58.48,9.65 58.48,9.88 58.41,9.96 58.17,9.96 58.14,9.98 58.14,10.74 57.99,10.9 57.61,10.9 57.45,10.74 57.45,10.06 57.38,9.98 57.15,9.98 57.07,10.06 57.07,10.74 56.92,10.9 54.03,10.9 53.42,10.29 52.58,10.29 v52.43,10.44 | U1.V16 40.75,8.52 40.69,8.46 40.69,7.77 v40.84,7.62
  Route15 0.076: v52.43,10.44 52.27,10.29 51.74,10.29 49.23,7.77 42.9,7.77 42.29,7.16 40.84,7.16 40.69,7.32 40.69,7.47 v40.84,7.62
CSI0_RXN1  (via drill 0.1 pad 0.25)
  Top 0.076: J4.5 63.25,9.61 63.25,10.44 63.48,10.67 63.48,10.97 63.4,11.05 63.17,11.05 63.09,10.97 63.09,10.76 63.02,10.68 62.79,10.68 62.71,10.76 62.71,10.97 62.64,11.05 62.41,11.05 62.33,10.97 62.33,10.87 62.18,10.72 61.8,10.72 61.65,10.87 61.65,10.97 61.57,11.05 53.95,11.05 53.65,10.74 53.03,10.74 v52.88,10.59 | v39.55,7.77 39.7,7.92 40.01,7.92 40.16,8.08 40.16,8.51 40.25,8.6 U1.V15
  Route15 0.076: v52.88,10.59 52.73,10.74 51.97,10.74 49.15,7.92 42.82,7.92 42.22,7.32 41.83,7.32 41.22,7.92 39.7,7.92 v39.55,7.77
CSI0_RXP0  (via drill 0.1 pad 0.25)
  Top 0.076: J4.3 60.88,9.25 60.88,8.46 60.66,8.23 60.66,7.85 60.5,7.7 59.66,7.7 59.21,8.15 58.22,8.15 57.99,8.38 57.99,10.67 57.91,10.74 57.68,10.74 57.61,10.67 57.61,9.98 57.45,9.83 57.07,9.83 56.92,9.98 56.92,10.67 56.84,10.74 54.1,10.74 53.49,10.13 52.58,10.13 v52.43,9.98 | v40.39,7.62 40.54,7.77 40.54,8.46 40.5,8.5 40.5,8.85 40.75,9.1 U1.U16
  Route15 0.076: v52.43,9.98 52.27,10.13 51.82,10.13 49.3,7.62 42.98,7.62 42.37,7.01 40.77,7.01 40.54,7.24 40.54,7.47 v40.39,7.62
CSI0_RXP1  (via drill 0.1 pad 0.25)
  Top 0.076: J4.6 63.86,9.59 63.86,10.44 63.63,10.67 63.63,11.05 63.48,11.2 62.33,11.2 62.18,11.05 62.18,10.95 62.1,10.87 61.87,10.87 61.8,10.95 61.8,11.05 61.65,11.2 53.87,11.2 53.57,10.9 53.03,10.9 v52.88,11.05 | v39.55,8.23 39.7,8.08 39.93,8.08 40.01,8.15 40.01,8.85 40.25,9.1 U1.U15
  Route15 0.076: v52.88,11.05 52.73,10.9 51.89,10.9 49.07,8.08 42.75,8.08 42.14,7.47 41.91,7.47 41.3,8.08 39.7,8.08 v39.55,8.23
EEPROM_WP
  Top 0.076: U4.5 74.73,16.76 79.4,16.76 79.63,16.99 79.63,18.75 81.92,21.03 81.92,21.95 82.45,22.48 84.58,22.48 85.11,23.01 85.11,25.07 85.42,25.38 91.47,25.38 J2.2
  Top 0.127: R7.1 94.23,23.57 93.67,24.13 J2.2
EMU0  (via drill 0.1 pad 0.25)
  Top 0.076: U1.D8 v36.5,16 | v22.4,19.2 23.32,20.12 23.32,20.8 21.18,22.94 18.36,22.94 17.68,23.62 R20.1
  Top 0.127: TC1.7 16.38,22.35 16.89,22.86 16.89,23.55 R20.1
  Bottom 0.076: v36.5,16 36.25,16.25 36.25,16.82 36.42,16.99 36.42,18.06 35.89,18.59 22.63,18.59 22.4,18.82 v22.4,19.2
EMU1  (via drill 0.1 pad 0.25)
  Top 0.076: U1.C8 v36.5,16.5 | v22.71,18.9 23.39,18.9 23.77,19.28 23.77,21.03 21.41,23.39 18.59,23.39 17.37,24.61 10.36,24.61 10.06,24.31 10.06,23.72 R21.1
  Top 0.127: R21.1 10.03,23.55 10.03,22.86 10.54,22.35 12.32,22.35 12.57,22.1 TC1.10
  Bottom 0.076: v22.71,18.9 22.86,18.75 35.97,18.75 36.6,18.11 36.6,16.94 36.5,16.84 v36.5,16.5
EXT_REFCLK1  (via drill 0.1 pad 0.25)
  Top 0.076: U1.D16 v41,16 | R56.1 1.68,5.18 1.83,5.03 4.95,5.03 v5.18,4.8
  Bottom 0.076: v41,16 41,15.88 39.88,14.75 37,14.75 36.58,14.33 33.91,14.33 32.54,15.7 32.54,16.99 31.93,17.6 23.09,17.6 21.57,16.08 21.57,14.48 20.19,13.11 15.93,13.11 15.16,12.34 15.16,5.94 14.48,5.26 10.97,5.26 10.67,4.95 5.33,4.95 v5.18,4.8
EXTINTN  (via drill 0.1 pad 0.25)
  Top 0.076: U1.C17 v41.5,16.5
  Top 0.127: U6.11 15.11,11.68 14.61,11.68 v14.35,11.94 R25.1
  Bottom 0.076: v41.5,16.5 U1.C17 40.88,16.25 40.75,16.38 40.75,17.77 38.02,20.5 22.63,20.5 20.34,18.21 20.34,16.31 19.81,15.77 15.32,15.77 15.09,15.54 15.09,12.95 14.35,12.22 v14.35,11.94
GND  (via drill 0.1 pad 0.25, 0.25 pad 0.46)
  Top 0.076: U1.H2 33.5,13.5 32.91,13.5 30.94,15.47 30.94,17.6 30.86,17.68 Y1.2 | R34.2 70.43,6.73 v69.98,6.73 | R29.2 v74.55,6.22 | R27.2 v76.58,6.22 | R26.2 v77.6,6.22 | U11.3 89.25,5.62 v89.38,5.49 | 30.35,19.58 30.43,19.66 31.01,19.66 31.24,19.43 31.24,15.62 32.85,14.01 33.35,14.01 33.59,14.25 U1.G2 34,14.5 v34,15 | U5.5 11.42,5.98 v11.18,6.22 | C18.2 13.64,8.94 v13.97,9.27 | U12.A1 33.16,24.75 v33.15,24.77 | U12.D1 | U12.D1 v33.15,23.24 | C61.2 33.52,22.66 U12.D1 | U13.A1 26.78,14.59 26.21,15.16 v26.21,15.39 | U13.D1 26.8,12.86 26.75,12.8 v26.75,12.57 | R76.1 37.47,22.84 v37.57,22.94 | R3.1 v37.47,25.27
  Top 0.127: v11.05,16.51 R35.1 | v11.05,13.46 R36.1 | TC1.5 v17.65,18.8 | TC1.3 v15.11,18.8 | R14.1 11.05,23.55 v11.05,22.86 | R37.2 v78.74,21.34 | R39.2 v76.71,21.34 | R40.2 v75.69,21.34 | R41.2 v74.68,21.34 | R42.2 v73.66,21.34 | J4.10 | J4.7 65.08,9.37 | Y1.2 30.13,17.68 29.84,17.4 28.88,17.4 C46.2 | 30.35,19.58 Y2.2 | v23.75,12.83 23.03,12.83 C53.2 | v23.75,13.46 24.23,13.46 | 24.23,13.46 24.34,13.46 C49.2 | C29.2 11.18,8.84 v11.18,8.26 | C50.2 11.43,14.86 11.56,14.99 R4.2 | v1.4,21.21 D1.2 | U4.2 v72.9,19.56 | v74.55,19.43 74.98,19.43 C35.2 | v75.82,18.41 75.23,18.41 C26.2 | v77.47,19.05 U8.2 | v79.63,13.08 C36.2 | D5.2 v84.71,15.49 | D4.2 v84.71,13.59 | D2.2 v84.71,11.68 | D3.2 v84.71,9.78 | v88.27,23.37 C58.2 | U9.4 10.28,14.23 10.14,14.1 8.76,14.1 v8.64,14.22 | U7.2 2,7.95 2.03,7.99 2.03,9.4 v1.78,9.65 | v3.94,6.22 3.94,5.71 R15.1 4.83,5.66 R6.1 | C34.2 v11.81,18.03 R63.2 | U5.5 12.2,6.02 13.61,6.02 C28.2 | 24.23,13.46 24.23,14.38 C14.2 24.23,14.43 24.23,15.22 C11.2 | C9.2 20.86,7.34 21.08,7.11 21.72,7.11 21.97,6.86 21.97,6.73 22.1,6.6 C5.2 | S1.P$4 25.1,7.7 C47.2 | C6.2 51.05,13.97 51.31,13.72 51.31,13.28 C22.2 | S1.P$3 25.91,11.92 C16.2 | C13.2 32.13,13.74 31.95,13.92 C10.2 31.62,14.15 v31.37,14.4 | v45.03,25.68 44.81,25.45 44.2,25.45 43.89,25.15 R1.1
  Top 0.152: U1.U1 v32.88,9.25 | U1.V2 v33.38,8.75 | U1.T3 v34,9.5 | U1.R3 v34,10 | U1.R4 v34.5,10 | U1.P4 v34.5,10.5 | U1.P5 v35,10.5 | U1.N5 v35,11 | U1.N6 v35.5,11 | U1.M6 v35.5,11.5 | U1.M7 v36,11.5 | U1.L7 v36,12 | U1.L8 v36.5,12 | U1.D3 v34,16 | U1.B1 v33,17 | U1.A2 v33.5,17.5 | U1.D4 v34.5,16 | U1.C4 v34.5,16.5 | U1.E6 v35.5,15.5 | U1.D14 v39.5,16 | U1.C14 v39.5,16.5 | U1.K8 v36.5,12.5 | U1.K9 v37,12.5 | U1.P16 v41,10.5 | U1.U19 v42.5,9 U1.V19 | U1.P21 v43.5,10.5 | v43.5,11 U1.N21 | U1.N22 v44,11 | U1.N23 v44.5,11 | U1.P24 v45,10.5 | U1.N24 v45,11 | U1.K15 v40.5,12.5 | U1.L19 v42.5,12 | U1.K19 v42.5,12.5 | U1.L20 v43,12 U1.M20 | U1.J14 v39.5,13.5 | U1.J15 v40.5,13.5 | U1.E20 v43,15.5 | U1.E21 v43.5,15.5 | U1.F20 v43,15 | U1.F21 v43.5,15 | U1.F23 v44.5,15 | U1.G20 v43,14.5 | U1.G23 v44.5,14.5 | U1.G24 v45,14.5 | U1.H24 v45,14 | U1.J24 v45,13.5 | U1.J19 v42.5,13.5 | U1.H19 v42.5,14 | U1.A27 v46.5,17.5 | U1.B28 v47.5,17.5 | v47,7.31 46.25,8.06 U1.V27 | v47,9 U1.U28 | U1.E10 v37.5,15.5 | U1.E12 v38.5,15.5 | U1.E13 v39,15.5 | U1.E18 v42,15.5 | U1.G19 v42.5,14.5 | U1.E19 v42.5,15.5 | U1.E22 v44,15.5 | U1.F22 v44,15 | U1.H20 v43,14 | U1.E23 v44.5,15.5 | U1.P19 v42.5,10.5 | U1.P20 v43,10.5 | U1.P22 v44,10.5 | U1.P23 v44.5,10.5 | U1.M24 v45,11.5 | U1.K14 v39.5,12.5 | U1.C3 v34,16.5 | U1.E9 v37,15.5 | U1.E11 v38,15.5 | U1.E3 v34,15.5 | U1.E4 v34.5,15.5 | U1.E5 v35,15.5 | U1.E7 v36,15.5 | U1.E8 v36.5,15.5 | U1.E16 v41,15.5 | U1.E17 v41.5,15.5 | U1.P3 v34,10.5 | U1.N3 v34,11 | U1.N4 v34.5,11 | U1.M4 v34.5,11.5 | U1.M5 v35,11.5 | U1.L5 v35,12 | U1.L6 v35.5,12 | U1.K6 v35.5,12.5 | U1.K7 v36,12.5 | U1.K20 v43,12.5 | U1.J20 v43,13.5 | U1.F19 v42.5,15 | U1.E24 v45,15.5 | U1.F24 v45,15 | U1.K24 v45,12.5 | U1.L24 v45,12 | U1.M23 v44.5,11.5 | U1.N20 v43,11 | U1.P17 v41.5,10.5 U1.P18 | U1.T19 v42.5,9.5
  Top 0.152: U1.B14 v39.5,17 U1.A14 39.75,17.58 39.93,17.75 40.31,17.75 40.44,17.88 C3.2 | C54.2 26.67,18.75 v28.12,17.3 28.63,17.3 C46.2 | v21.95,5.77 21.84,5.87 C17.2 | C5.2 22.48,6.55 v22.48,5.77 | C4.2 29.72,9.63 v30.02,9.93 30.48,9.47 C1.2 | U1.G2 U1.H2 | C19.2 40.56,6.73 v40.62,6.78 40.67,6.73 C2.2 | C15.2 C8.2 C20.2 v29.51,11.13 v29.52,11.12 | C12.2 27.86,14.15 v27.61,14.4 | C63.2 v39.12,20.95 | 38.56,20.45 v39.12,20.45
  Top 0.254: U9.4 11.37,14.49 C50.2 | U6.15 14.75,9.67 14.35,9.27 v13.97,9.27 | C42.2 v15.11,16.97 | C40.2 v16.13,16.97 | C51.2 v17.14,16.97 | C52.2 v18.16,16.97 | C45.2 v19.81,5.31 | C39.2 18.8,5.56 v18.54,5.31 | C44.2 v17.78,5.31 | C38.2 v16.76,5.31 | v16,5.31 15.75,5.56 C43.2 | X1.G0 100.35,21.7 100.33,21.69 v100.33,20.7 | X1.G1 99.43,8.76 v100.71,8.76 | C29.2 11.12,8.97 12.06,9.91 C41.2 | v97.92,11.68 X1.PIN6 | J4.10 v68.05,8.08 | 65.08,9.37 v65.08,8.08 | v62.71,8.08 62.33,8.08 62.04,8.37 J4.4 | J4.1 59.05,9.42 v59.05,10.67 | J6.A1 63.29,19.73 v63.12,19.56 63.29,19.39 J6.B12 | J6.A12 68.79,19.73 v68.96,19.56 68.79,19.39 J6.B1 | U2.4 60.67,17.86 C24.2 60.71,17.78 v60.71,17.14 | C37.2 v78.36,13.59 | v88.9,24.64 C57.2 | C23.2 51.31,12.01 v51.31,12.57 51.31,13.13 C22.2 | C16.2 25.83,13.21 24.68,13.21 C49.2 | C55.2 v7.49,24.64 | v2.41,24.64 C59.2 | C56.2 v8,23.37 | C60.2 8.46,20.02 8.26,19.81 v8.26,19.56 | C21.2 38.56,20.09 38.56,20.45 C63.2
  Top 0.381: J5.SH3_B v1.27,10.92 | J5.B1_A12 7.38,12.06 v8.26,12.06 8.51,12.32 9.06,12.32 C32.2 | J5.A1_B12 7.38,18.41 v8.38,18.41 | J5.SH1_T v8.26,19.56 | v1.27,19.56 J5.SH4_T | J5.SH2_B v8.26,10.92 8.93,10.92 C31.2 | J6.SH_B_1 v62.48,21.72 | J6.SH_B_4 v62.48,17.4 | v69.6,17.4 J6.SH_T_3 | J6.SH_T_2 v67.39,21.72
  Top 0.508: U10.2 83.44,25.78 JP4.33
  Bottom 0.152: v22.48,5.77 22.48,5.87 | v21.95,5.77 19.99,3.81 JP3.8 | J8.6 21.95,6.48 21.95,5.87 | 21.95,5.87 v21.95,5.77 | 22.4,5.79 22.45,5.79 v22.48,5.77 | 22.4,5.79 22.02,5.79 | 22.02,5.79 21.97,5.79 v21.95,5.77 | v22.48,5.77 22.5,5.79 22.55,5.79 | 38.94,6.17 38.94,5.94 38.79,5.79 37.57,5.79 | 22.55,5.79 23.85,5.79 | 23.93,5.79 23.85,5.79 | 25.45,5.79 25.38,5.79 | 25.38,5.79 24,5.79 | 24,5.79 23.93,5.79 | 25.45,5.79 25.53,5.79 | 25.53,5.79 26.9,5.79 | 26.9,5.79 26.98,5.79 | 26.98,5.79 27.05,5.79 | 27.05,5.79 28.35,5.79 | 28.35,5.79 28.42,5.79 | 28.42,5.79 28.5,5.79 | 28.5,5.79 29.87,5.79 | 29.87,5.79 29.95,5.79 | 29.95,5.79 30.02,5.79 | 30.02,5.79 31.39,5.79 | 31.39,5.79 31.47,5.79 | 31.47,5.79 31.55,5.79 | 31.55,5.79 32.84,5.79 | 32.84,5.79 32.92,5.79 | 32.92,5.79 32.99,5.79 | 32.99,5.79 34.37,5.79 | 34.37,5.79 34.44,5.79 | 34.44,5.79 34.52,5.79 | 34.52,5.79 35.89,5.79 | 35.89,5.79 35.97,5.79 | 35.97,5.79 36.04,5.79 | 36.04,5.79 37.41,5.79 | 37.41,5.79 37.49,5.79 | 37.49,5.79 37.57,5.79 | J8.37 37.49,6.46 37.49,5.87 | 37.49,5.87 37.49,5.79 | J8.34 35.97,5.87 | 35.97,5.87 35.97,5.79 | J8.31 34.44,6.47 34.44,5.87 | 34.44,5.87 34.44,5.79 | J8.28 32.92,6.45 32.92,5.87 | 32.92,5.87 32.92,5.79 | J8.25 31.47,5.87 | 31.47,5.87 31.47,5.79 | J8.22 29.95,6.48 29.95,5.87 | 29.95,5.87 29.95,5.79 | J8.19 28.42,6.45 28.42,5.87 | 28.42,5.87 28.42,5.79 | J8.16 26.98,6.48 26.98,5.87 | 26.98,5.87 26.98,5.79 | J8.13 25.45,5.87 | 25.45,5.87 25.45,5.79 | J8.10 23.93,6.46 23.93,5.87 | 23.93,5.87 23.93,5.79 | 23.85,5.79 23.93,5.87 | 24,5.79 23.93,5.87 | 22.4,5.79 22.48,5.87 | 22.55,5.79 22.48,5.87 | 22.02,5.79 21.95,5.87 | 25.38,5.79 25.45,5.87 | 25.53,5.79 25.45,5.87 | 26.9,5.79 26.98,5.87 | 27.05,5.79 26.98,5.87
  Bottom 0.152: 28.35,5.79 28.42,5.87 | 28.5,5.79 28.42,5.87 | 29.87,5.79 29.95,5.87 | 30.02,5.79 29.95,5.87 | 31.39,5.79 31.47,5.87 | 31.55,5.79 31.47,5.87 | 32.84,5.79 32.92,5.87 | 32.99,5.79 32.92,5.87 | 34.37,5.79 34.44,5.87 | 34.52,5.79 34.44,5.87 | 35.89,5.79 35.97,5.87 | 36.04,5.79 35.97,5.87 | 37.41,5.79 37.49,5.87 | 37.57,5.79 37.49,5.87 | J8.7 22.48,6.47 22.48,5.87
  Bottom 0.254: v41.5,10.5 v41,10.5 41,9.42 41.23,9.19 J8.S2 | v40.62,6.78 40.23,6.4 39.17,6.4 | 38.94,6.17 39.17,6.4 | J8.S1 16.72,9.19 16.38,9.53 v16.38,10.54 | 39.17,6.4 39.05,6.4 J8.40 | 39.17,6.4 38.94,6.63
  Bottom 0.381: v1.27,10.92 J5.SH3_B | v8.26,19.56 J5.SH1_T | J5.SH4_T v1.27,19.56 | v8.26,10.92 v8.25,10.92 J5.SH2_B | v62.48,21.72 J6.SH_B_1 | v62.48,17.4 J6.SH_B_4 | v69.6,17.4 J6.SH_T_3 | J6.SH_T_2 v67.39,21.72
  other vias: 11.18,7.24 18.67,12.06 16.38,12.06 18.67,10.54 17.53,10.92 79.88,6.22 79.88,7.49 79.88,6.86 5.71,7.95 6.1,7.95 6.48,7.95 5.71,7.57 6.1,7.57 6.48,7.57 6.48,8.33 6.1,8.33 5.71,8.33 23.09,8.23 23.47,8.23 23.85,8.61 23.85,8.23 40.13,24.13 40.51,24.13 40.89,24.13 40.13,23.75 40.13,23.37
  pour Route2 (isolate 0.127, rank 6): -5.08,35.56 106.68,35.56 106.68,-5.08 -5.08,-5.08
  pour Top (no thermals): 7.49,8.76 6.48,8.76 6.48,8.38 4.45,8.38 4.45,7.24 7.87,7.24 7.87,8.13 7.49,8.13
  pour Top (no thermals): 11.43,9.27 10.92,9.27 10.92,5.84 12.45,5.84 12.45,6.1 11.43,6.1
  pour Top (no thermals): 25.15,13.72 25.15,12.45 22.23,12.45 22.23,13.72
  pour Top (no thermals): 79.5,7.8 79.5,5.21 82.42,5.21 82.42,7.8
  pour Top (no thermals): 22.23,8.89 25.15,8.89 25.15,7.49 23.11,7.49 23.11,8.13 22.73,8.13 22.48,8.38 22.23,8.38
  pour Bottom (isolate 0.127, rank 6): -2.54,-2.54 104.14,-2.54 104.14,33.02 -2.54,33.02
  pour Top (no thermals): 41.02,25.02 41.02,23.11 39.88,23.11 39.88,25.02
GPMC0_AD0  (via drill 0.1 pad 0.25)
  Top 0.076: v47.55,14.1 47.17,14.1 47.02,14.25 U1.G28 | v71.6,23.85 71.6,23.19 R51.1
  Bottom 0.076: v47.55,14.1 48.39,13.26 50.52,13.26 53.49,16.23 53.49,20.42 54.18,21.11 57.07,21.11 58.14,22.17 61.42,22.17 62.03,22.78 70.33,22.78 71.4,23.85 v71.6,23.85 71.75,23.7 83.97,23.7 86.49,26.21 86.49,27.13 87.02,27.66 96.32,27.66 97.79,29.13 JP5.39
GPMC0_AD1  (via drill 0.1 pad 0.25)
  Top 0.076: U1.G27 46.5,14.5 47.53,14.5 v47.55,14.48 | v72.59,24 72.64,23.95 R49.1
  Bottom 0.076: v47.55,14.48 48.62,13.41 50.44,13.41 53.34,16.31 53.34,20.5 54.1,21.26 57,21.26 58.06,22.33 61.34,22.33 61.95,22.94 70.26,22.94 71.48,24.16 72.44,24.16 v72.59,24 72.75,23.85 83.9,23.85 86.33,26.29 86.33,27.2 86.94,27.81 93.88,27.81 95.25,29.18 JP5.38
GPMC0_AD2  (via drill 0.1 pad 0.25)
  Top 0.076: v47.93,14.48 47.66,14.75 U1.F28 | v73.58,24.16 73.58,23.24 R42.1
  Bottom 0.076: v47.93,14.48 48.84,13.56 50.37,13.56 53.19,16.38 53.19,20.57 54.03,21.41 56.92,21.41 57.99,22.48 61.27,22.48 61.87,23.09 70.18,23.09 71.4,24.31 73.43,24.31 v73.58,24.16 73.74,24 83.82,24 86.18,26.36 86.18,27.3 86.84,27.96 91.52,27.96 92.71,29.16 JP5.37
GPMC0_AD3  (via drill 0.1 pad 0.25)
  Top 0.076: U1.F27 46.5,15 47.79,15 v48.31,14.48 | v74.57,24.31 74.57,23.27 R41.1
  Bottom 0.076: v48.31,14.48 49.07,13.72 50.29,13.72 53.03,16.46 53.03,20.65 53.95,21.57 56.84,21.57 57.91,22.63 61.19,22.63 61.8,23.24 70.1,23.24 71.32,24.46 74.42,24.46 v74.57,24.31 74.73,24.16 82.36,24.16 84.12,25.92 84.12,27.66 84.58,28.12 89.08,28.12 JP5.36
GPMC0_AD4  (via drill 0.1 pad 0.25)
  Top 0.076: v48.69,14.48 47.92,15.25 U1.E28 | v75.64,24.46 75.69,24.41 R40.1
  Bottom 0.076: v48.69,14.48 49.3,13.87 50.22,13.87 52.88,16.54 52.88,20.73 53.87,21.72 56.77,21.72 57.84,22.78 61.11,22.78 61.72,23.39 70.03,23.39 71.25,24.61 75.49,24.61 v75.64,24.46 75.79,24.31 82.3,24.31 83.97,25.98 83.97,27.74 84.51,28.27 85.65,28.27 86.59,29.21 JP5.35
GPMC0_AD5  (via drill 0.1 pad 0.25)
  Top 0.076: U1.E27 46.5,15.5 48.05,15.5 v49.07,14.48 | R39.1 76.58,23.29 v76.58,24.61
  Bottom 0.076: v49.07,14.48 49.53,14.02 50.14,14.02 52.73,16.61 52.73,20.8 53.8,21.87 56.69,21.87 57.76,22.94 61.04,22.94 61.65,23.55 69.95,23.55 71.17,24.77 76.43,24.77 v76.58,24.61 76.73,24.46 82.22,24.46 83.82,26.06 83.82,27.96 85.06,29.21 JP5.34
GPMC0_AD6  (via drill 0.1 pad 0.25)
  Top 0.076: v49.45,14.48 48.23,15.7 47.09,15.7 47.04,15.75 U1.D28 | v76.96,24.77 76.96,23.93 R38.1
  Bottom 0.076: v49.45,14.48 49.76,14.17 50.06,14.17 52.58,16.69 52.58,20.88 53.72,22.02 56.62,22.02 57.68,23.09 60.96,23.09 61.57,23.7 69.88,23.7 71.09,24.92 76.81,24.92 v76.96,24.77 77.11,24.61 82.14,24.61 83.67,26.14 83.67,28.09 JP5.33
GPMC0_AD7  (via drill 0.1 pad 0.25)
  Top 0.076: v49.84,14.48 48.46,15.85 47.24,15.85 47.09,16 46.5,16 U1.D27 | R37.1 77.34,24.56 v77.34,24.92
  Bottom 0.076: v49.84,14.48 50.14,14.48 52.43,16.76 52.43,20.95 53.65,22.17 56.54,22.17 57.61,23.24 60.88,23.24 61.49,23.85 69.8,23.85 71.02,25.07 77.19,25.07 v77.34,24.92 77.5,24.77 79.93,24.77 81.23,26.06 81.23,28.04 80.06,29.21 JP5.32
GPMC0_AD8
  Top 0.076: U1.L27 46.5,12 47.44,12 52.96,6.48 58.37,6.48 58.83,6.02 69.72,6.02 70.08,5.66 R34.1 70.48,4.88 71.09,4.27 71.09,2.56 JP2.29
GPMC0_AD9
  Top 0.076: U1.L28 47.41,12.25 53.03,6.63 58.45,6.63 58.9,6.17 70.84,6.17 70.99,6.02 70.99,5.84 71.2,5.64 71.5,5.64 | R32.1 71.5,5.64 | 71.5,5.64 71.5,4.7 JP3.29
GPMC0_AD10
  Top 0.076: U1.K27 46.5,12.5 47.39,12.5 53.11,6.78 58.52,6.78 58.98,6.33 68.81,6.33 69.72,7.24 71.86,7.24 72.01,7.09 72.01,5.84 72.19,5.66 R31.1 72.52,5.28 73.69,4.12 73.69,2.52 JP2.30
GPMC0_AD11
  Top 0.076: U1.K28 47.37,12.75 53.19,6.93 58.6,6.93 59.05,6.48 68.73,6.48 69.65,7.39 72.77,7.39 73.03,7.14 73.03,5.84 73.2,5.66 R30.1 73.53,5.21 JP3.30
GPMC0_AD12
  Top 0.076: U1.J28 47.1,13.25 53.26,7.09 58.67,7.09 59.13,6.63 68.66,6.63 69.57,7.54 73.61,7.54 74.04,7.11 74.04,5.84 74.22,5.66 R29.1 74.55,5.08 74.83,4.8 75.51,4.8 76.12,4.19 76.12,2.62 JP2.31
GPMC0_AD13
  Top 0.076: U1.J27 46.5,13.5 47.08,13.5 53.34,7.24 58.75,7.24 59.21,6.78 68.58,6.78 69.49,7.7 74.45,7.7 75.06,7.09 75.06,5.84 75.23,5.66 R28.1 75.56,5.13 75.89,4.8 76.48,4.8 JP3.31
GPMC0_AD14
  Top 0.076: U1.H28 47.06,13.75 53.42,7.39 58.83,7.39 59.28,6.93 68.5,6.93 69.42,7.85 75.36,7.85 76.07,7.14 76.07,5.84 76.25,5.66 R27.1 76.58,5.11 76.81,4.88 78.33,4.88 78.79,4.42 78.79,2.49 JP2.32
GPMC0_AD15
  Top 0.076: U1.H27 46.5,14 47.04,14 53.49,7.54 58.9,7.54 59.36,7.09 68.43,7.09 69.34,8 76.2,8 77.09,7.11 77.09,5.84 77.27,5.66 R26.1 77.6,5.23 77.8,5.03 78.72,5.03 79.93,3.81 JP3.32
GPMC0_ADVN_ALE  (via drill 0.1 pad 0.25)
